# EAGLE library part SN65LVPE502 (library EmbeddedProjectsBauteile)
Texas Instruments Dual Channel USB3.0 Redriver/Equalizer
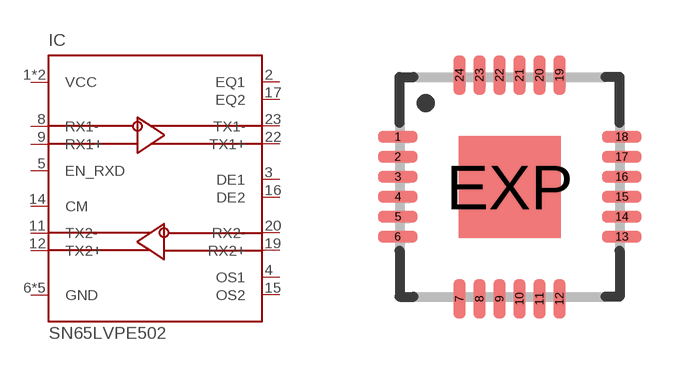
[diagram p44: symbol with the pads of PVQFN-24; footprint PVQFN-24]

Designator prefix IC

## SN65LVPE502RGET (EP: 401344)  [PVQFN-24]
1  VCC  pwr
2  EQ1
3  DE1
4  OS1
5  EN_RXD  in
6  GND  pwr
8  RX1-  in
9  RX1+  in
10  GND  pwr
11  TX2-  out
12  TX2+  out
13  VCC  pwr
14  CM
15  OS2
16  DE2
17  EQ2
18  GND  pwr
19  RX2+  in
20  RX2-  in
21  GND  pwr
22  TX1+  out
23  TX1-  out
EXP  GND  pwr

## Footprint PVQFN-24 (pad centres in mm)
smd 1 x 0.3: 1 -2.8,1.25; 2 -2.8,0.75; 3 -2.8,0.25; 4 -2.8,-0.25; 5 -2.8,-0.75; 6 -2.8,-1.25; 13 2.8,-1.25; 14 2.8,-0.75; 15 2.8,-0.25; 16 2.8,0.25; 17 2.8,0.75; 18 2.8,1.25
smd 0.3 x 1: 7 -1.25,-2.8; 8 -0.75,-2.8; 9 -0.25,-2.8; 10 0.25,-2.8; 11 0.75,-2.8; 12 1.25,-2.8; 19 1.25,2.8; 20 0.75,2.8; 21 0.25,2.8; 22 -0.25,2.8; 23 -0.75,2.8; 24 -1.25,2.8
smd 2.54 x 2.54: EXP 0,0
